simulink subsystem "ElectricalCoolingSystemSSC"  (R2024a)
settings: Solver=VariableStepAuto  StartTime=0.0  StopTime=10.0  RelTol=1e-3
undefined symbols (not defined in the file): BattTempInit, One, Pass, pipe, pump, radiator, T_env, tank, ThrmBatt1, ThrmBatt2, ThrmBatt3, ThrmBatt4, ThrmEM1, ThrmEM2, ThrmEM3, ThrmEM4, valve
libraries: fl_lib x109, SimscapeFluids_lib x7, nesl_utility_internal x6, autolibutils x2, nesl_utility x1, sdl_lib x1
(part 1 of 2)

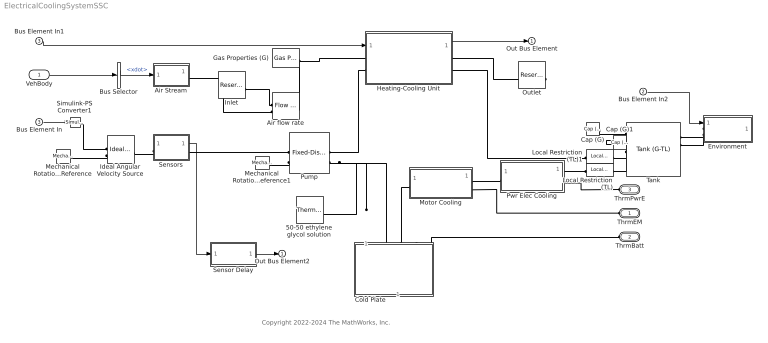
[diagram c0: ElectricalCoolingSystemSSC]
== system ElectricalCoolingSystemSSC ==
  note: Copyright 2022-2024 The MathWorks, Inc.
  VehBody : Inport
  Bus Element In2 : Inport  Port=2
  Bus Element In1 : Inport  Port=3
  Bus Element In : Inport  Port=3
  50-50 ethylene glycol solution : SimscapeFluids_lib/Thermal Liquid/Utilities/Thermal Liquid Properties (TL)  fluid_list=fluids.thermal_liquid.utilities.enum.thermal_liquid_fluid_list.ethylene_glycol  concentration_param_EG=fluids.thermal_liquid.utilities.enum.thermal_liquid_concentration.volume_fraction  concentration_param_PG=fluids.thermal_liquid.utilities.enum.thermal_liquid_concentration.volume_fraction  c_mass_SW=3.5e-3  c_mass_EG=0.1  c_mass_PG=0.1  c_mass_GL=0.1  c_vol_EG=0.5  c_vol_PG=0.1  beta_const_EG=2.1791 GPa  beta_const_PG=2.1791 GPa  beta_const_GL=2.1791 GPa  p_min_EG=0.01 MPa  p_min_PG=0.01 MPa  p_min_GL=0.01 MPa  p_max_EG=50 MPa  p_max_PG=50 MPa  p_max_GL=50 MPa  p_atm=0.101325 MPa  properties_range_check=simscape.enum.assert.action.error
  Air Stream : Subsystem
  Air flow rate : fl_lib/Gas/Sources/Flow Rate Source (G)  source_type=foundation.enum.constant_controlled.controlled  flow_type=foundation.enum.mass_volumetric_flow.mass  mass_flow=0 kg/s  volumetric_flow=0 m^3/s  volumetric_flow_conditions=foundation.enum.volumetric_flow_conditions.actual  p_std=0.101325 MPa  T_std=20 degC  power_spec=0  area_A=radiator.area_air m^2  area_B=radiator.area_air m^2
  Bus Selector : BusSelector  OutputSignals=BdyFrm.Cg.Vel.xdot
  Cap (G) : fl_lib/Gas/Elements/Cap (G)  p_specify=off  p_priority=None  p=0.101325 MPa  p_nominal_specify=off  p_nominal_value=1  p_nominal_unit=MPa  T_specify=off  T_priority=None  T=293.15 K  T_nominal_specify=off  T_nominal_value=1  T_nominal_unit=K
  Cap (G)1 : fl_lib/Gas/Elements/Cap (G)  p_specify=off  p_priority=None  p=0.101325 MPa  p_nominal_specify=off  p_nominal_value=1  p_nominal_unit=MPa  T_specify=off  T_priority=None  T=293.15 K  T_nominal_specify=off  T_nominal_value=1  T_nominal_unit=K
  Cold Plate : Subsystem  Variant=on  VariantControlMode=label  VariantControl=Choice  LabelModeActiveChoice=One-Pass
  Environment : Subsystem
  Gas Properties (G) : fl_lib/Gas/Utilities/Gas Properties (G)  gas_spec=1  R=0.287 kJ/kg/K  Z=1  T_ref=293.15 K  h_ref=420 kJ/kg  cp_ref=1 kJ/kg/K  mu_ref=18 s*uPa  k_ref=26 mW/m/K  T_TLU1=[150 : 10 : 200, 250 : 50 : 1000, 1500, 2000] K  h_TLU1=[275.264783730547; 285.377054177734; 295.474578903607; 305.560871069627; 315.638490783961; 325.709373787179; 376.008033649461; 426.297784741196; 476.678788323875; 527.253890684429; 578.12722735187; 629.395040865183; 681.137690131207; 733.415442873049; 786.267894376777; 839.715851152006; 893.764459999509; 948.406676876931; 1003.62653219711; 1059.40193232821; 1115.70691941005; 1172.51341226958; 1762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  cp_TLU1=[1.01211492398124; 1.01042105529234; 1.00914159006373; 1.00815898273273; 1.00739688341918; 1.00680484569075; 1.00554191216852; 1.00637389921747; 1.0092105862442; 1.01414404435034; 1.02111299587909; 1.02986878923959; 1.04003820504128; 1.05120320041448; 1.06296312852444; 1.07497111709439; 1.08694865668905; 1.0986858495625; 1.11003396604319; 1.12089493621399; 1.13121051694521; 1.14095251451866; 1.210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  mu_TLU1=[10.3766056544352; 10.9908682444892; 11.5932000841352; 12.1841060353213; 12.764067709023; 13.3335437107148; 16.038149065057; 18.5373404836509; 20.8671495114253; 23.0554226800681; 25.1239717991959; 27.0901379793485; 28.96790749834; 30.7687111230031; 32.5020036481173; 34.17569027566; 35.7964450415303; 37.3699520751368; 38.9010908824946; 40.3940804368247; 41.8525925389218; 43.279841956487; 56.3254722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  k_TLU1=[14.1517155766309; 15.0474512994325; 15.9300520513026; 16.7998749295306; 17.6573089963228; 18.5027588910197; 22.5644026699512; 26.384465676638; 30.0032801168886; 33.4532006033488; 36.7600619429332; 39.9446251241844; 43.0237448740114; 46.0112537033799; 48.9186234516389; 51.7554617696538; 54.5298878921773; 57.2488200454925; 59.9181976996146; 62.5431553064749; 65.128159527924; 67.6771186900213; 91.78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  T_TLU2=[150 : 10 : 200, 250 : 50 : 1000, 1500, 2000] K  p_TLU2=[0.001, 0.005, 0.01 : 0.01 : 0.1, 0.12, 0.15, 0.2, 0.5, 1, 2, 5, 10] MPa  rho_TLU2=[.0232262435294122, .116159536418799, .232389928446798, .465063671432694, .698022015548056, .931265751213184, 1.16479567270147, 1.39861257816015, 1.6327172696322, 1.86711055307826, 2.10179323839862, 2.33676613945539, 2.80758586416975, 3.5160126461103, 4.70263894299404, 11.983516436453, 24.7878864888476, 53.4753944012435, 188.202476404452, 488.088746553617; .0217743613495483, .108893511712, .217841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  s_TLU2=[4.51795188269071, 4.05581817155212, 3.85666832168988, 3.65733557342939, 3.54058125651975, 3.45763599951791, 3.39321600973057, 3.34051347760226, 3.2958969095816, 3.25719862711102, 3.22302043260479, 3.19240764614444, 3.13933271586112, 3.07416650003008, 2.98972303348322, 2.71525667312277, 2.4961408855038, 2.25200576011077, 1.78471429674036, 1.29090458888978; 4.58264139768585, 4.12053027678858, 3.921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  h_TLU2=[276.08088424589, 276.048494255671, 276.007989595737, 275.926922934925, 275.845779642901, 275.764559507019, 275.68326231383, 275.601887849085, 275.520435897725, 275.438906243879, 275.357298670861, 275.275612961165, 275.112006257597, 274.86600469197, 274.45440990197, 271.941510053176, 267.573991878308, 258.028969756929, 218.234362269026, 158.930370089034; 286.104280121225, 286.075386875978, 286.039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  cp_TLU2=[1.00234082589656, 1.00272486727657, 1.00320557010184, 1.0041691525775, 1.00513564892549, 1.00610507294701, 1.00707743852905, 1.00805275964505, 1.00903105035552, 1.01001232480866, 1.01099659724104, 1.01198388197822, 1.01396754611819, 1.01696599794404, 1.02202562270308, 1.05412155485561, 1.1152747482059, 1.27776397304517, 2.72714600163742, 2.84169679152775; 1.00233987250094, 1.0026582461868, 1.0030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  mu_TLU2=[10.3589401268092, 10.3596215490306, 10.3604759816291, 10.3621937105615, 10.3639232830336, 10.3656647294411, 10.367418080323, 10.3691833663632, 10.3709606183908, 10.3727498673813, 10.3745511444581, 10.3763644808926, 10.3800274576703, 10.3856131584654, 10.3951680979376, 10.4591651061333, 10.5933716881858, 10.987254253246, 14.2772531553238, 32.0640438449792; 10.9730737505367, 10.9737639649823, 10.97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  k_TLU2=[14.0836394676256, 14.0862942007498, 14.0896194596466, 14.0962928994967, 14.102997040872, 14.1097320212018, 14.1164979631452, 14.1232949816993, 14.1301231872323, 14.1369826870758, 14.143873586467, 14.1507959891554, 14.1647357143434, 14.1858841226196, 14.2217750346856, 14.4546939871274, 14.9161812046845, 16.179147415959, 25.804405174674, 52.7180018225101; 14.9842167167395, 14.9866891286677, 14.9897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  beta_TLU2=[.000999939063271047, .00499847620325299, .00999390291790365, .019975596477506, .0299450577879351, .0399022638252297, .0498471914323395, .0597798173190184, .0697001180617656, .0796080701037593, .0895036497547952, .0993868331912267, .119115915458133, .148615963978671, .197531539031374, .484259268054388, .934728751330763, 1.71724988255064, 2.82175958388315, 17.9919018393343; .000999950175637603, .00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  alpha_TLU2=[.00666792026017809, .00667293852525301, .00667922012518017, .00669181264110188, .00670444439920956, .0067171155853866, .00672982638662978, .00674257699105705, .00675536758791526, .00676819836758812, .00678106952160409, .00679398124264439, .00681992716233515, .00685915517876874, .00692537286982025, .00734607851757868, .00815022150220267, .0102947700145685, .0286130234990625, .0187953609548895; .00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  T_min_perfect=1 K  T_max_perfect=inf K  p_min_perfect=1e-6 MPa  p_max_perfect=inf MPa  T_range_flag=1  T_min_semiperfect=150 K  T_max_semiperfect=2000 K  p_min_semiperfect=1e-6 MPa  p_max_semiperfect=inf MPa  pT_region_flag=1  pT_validity_TLU2=ones(24, 20)  T_min_real=150 K  T_max_real=2000 K  p_min_real=0.001 MPa  p_max_real=10 MPa  p_atm=0.101325 MPa  properties_range_check=simscape.enum.assert.action.error  Mach_rev=0.001
  Heating-Cooling Unit : Subsystem
  Ideal Angular Velocity Source : fl_lib/Mechanical/Mechanical Sources/Ideal Angular Velocity Source
  Inlet : fl_lib/Gas/Elements/Reservoir (G)  pressure_spec=1  reservoir_pressure=0.101325 MPa  reservoir_temperature=EnvAirTempC degC  area_A=radiator.area_air m^2
  Local Restriction (TL) : fl_lib/Thermal Liquid/Elements/Local Restriction (TL)  restriction_type=foundation.enum.restriction_type.fixed  restriction_area=pipe.area/1.1 cm^2  min_area=1e-10 m^2  max_area=0.005 m^2  area=pipe.area cm^2  Cd=0.7  Re_c=12  pressure_recovery=simscape.enum.onoff.on
  Local Restriction (TL)1 : fl_lib/Thermal Liquid/Elements/Local Restriction (TL)  restriction_type=foundation.enum.restriction_type.fixed  restriction_area=pipe.area/1.1 cm^2  min_area=1e-10 m^2  max_area=0.005 m^2  area=pipe.area cm^2  Cd=0.7  Re_c=12  pressure_recovery=simscape.enum.onoff.on
  Mechanical Rotational Reference : fl_lib/Mechanical/Rotational Elements/Mechanical Rotational Reference
  Mechanical Rotational Reference1 : fl_lib/Mechanical/Rotational Elements/Mechanical Rotational Reference
  Motor Cooling : Subsystem  Tag=PublishSubsystem
  Outlet : fl_lib/Gas/Elements/Reservoir (G)  pressure_spec=1  reservoir_pressure=0.101325 MPa  reservoir_temperature=EnvAirTempC K  area_A=radiator.area_air m^2
  Pump : SimscapeFluids_lib/Thermal Liquid/Pumps & Motors/Fixed-Displacement Pump (TL)  loss_spec=1  displacement=pump.displacement cm^3/rev  omega_nominal=pump.omega rpm  p_nominal=1 MPa  mu_nominal=0.9 cP  vol_eff_nominal=0.92  mech_eff_nominal=1/(1 + (0.6)/(pump.displacement)*6.283185307179584 + (0.05)/(pump.displacement)/(1)*6.283185307179584)  no_load_torque=0.05 N*m  p_diff_eff_TLU=[.1, 1, 2] MPa  omega_eff_TLU=[25, 50, 100, 200, 300, 400] rad/s  vol_eff_TLU=[.816, .908, .954, .977, .981, .984; .325, .663, .831, .916, .925, .946; .137, .568, .78, .892, .893, .91]  mech_eff_TLU=[.996, .996, .996, .996, .996, .996; .988, .989, .989, .989, .989, .99; .981, .981, .982, .982, .983, .984]  p_diff_loss_TLU=[.1, 1, 2] MPa  omega_loss_TLU=[25, 50, 100, 200, 300, 400] rad/s  vol_loss_TLU=[.023, .023, .023, .023, .0285, .032; .0844, .0842, .0845, .084, .1125, .108; .1079, .108, .11, .108, .1605, .18] * 1e-3 m^3/s  mech_loss_TLU=[.002, .002, .002, .002, .002, .002; .0607, .0556, .0556, .0556, .0556, .0505; .1937, .1937, .1833, .1833, .1729, .1626] N*m  vol_eff_min=1e-3  vol_eff_max=1  mech_eff_min=1e-3  mech_eff_max=1  pressure_threshold=1e-3 MPa  omega_threshold=10 rad/s  area=pipe.area cm^2  supplied_range_check=0  pump_mode_check=simscape.enum.assert.action.none
  Pwr Elec Cooling : Subsystem
  Sensor Delay : Subsystem  mask{wc=10, InitCond=0, dataType=off}
      mask prompts: wc "Cutoff frequency, wc [rad/s]"; InitCond "Initial condition, InitCond [same as u]"; dataType "Enforce same input data type"
  Sensors : Subsystem
  Simulink-PS Converter1 : nesl_utility_internal/Simulink-PS Converter  PhysicalDomain=network_engine_domain  SubClassName=ps_input  LeftPortType=input  RightPortType=output  PseudoPeriodic=off  Frequencies=[]  NoiseDistribution=none  NoiseParameters=[]  Unit=rpm  AffineConversion=off  FilteringAndDerivatives=provide  SimscapeFilterOrder=1  InputFilterTimeConstant=0.001  UdotUserProvided=0
  Tank : SimscapeFluids_lib/Thermal Liquid/Tanks & Accumulators/Tank (G-TL)  num_inlet=6  volume_total=tank.volume l  volume_spec=1  tank_area=tank.area m^2  level_TLU=[0, 3, 5] m  volume_TLU=[0, 4, 6] m^3  inlet_areas_A1B1=[.01, .01] m^2  inlet_height_A2=0.1 m  inlet_area_A2=0.01 m^2  inlet_heights_A2B2=[0.0, 0.0] m  inlet_areas_A2B2=pipe.area*[1.0, 1.0] cm^2  inlet_heights_A2B2C2=[.1, .05, 0] m  inlet_areas_A2B2C2=[.01, .01, .01] m^2  inlet_heights_A2B2C2D2=0.1 * ones(1, 4) m  inlet_areas_A2B2C2D2=0.01 * ones(1, 4) m^2  inlet_heights_A2B2C2D2E2=0.1 * ones(1, 5) m  inlet_areas_A2B2C2D2E2=0.01 * ones(1, 5) m^2  inlet_heights_A2B2C2D2E2F2=0.07 * ones(1, 6) m  inlet_areas_A2B2C2D2E2F2=0.01 * ones(1, 6) m^2  capacity_check=1  max_liquid_capacity=tank.volume l  g=0 m/s^2  level_specify=on  level_priority=None  level=0.2 m  level_nominal_specify=off  level_nominal_value=1  level_nominal_unit=m  volume_liquid_specify=on  volume_liquid_priority=High  volume_liquid=5 l  volume_liquid_nominal_specify=off  volume_liquid_nominal_value=1  volume_liquid_nominal_unit=m^3  mass_liquid_specify=off  mass_liquid_priority=None  mass_liquid=5e+3 kg  mass_liquid_nominal_specify=off  mass_liquid_nominal_value=1  mass_liquid_nominal_unit=kg  T_liquid_specify=off  T_liquid_priority=High  T_liquid=293.15 K  T_liquid_nominal_specify=off  T_liquid_nominal_value=1  T_liquid_nominal_unit=K  p_gas_specify=off  p_gas_priority=High  p_gas=0.101325 MPa  p_gas_nominal_specify=off  p_gas_nominal_value=1  p_gas_nominal_unit=MPa  T_gas_specify=off  T_gas_priority=High  T_gas=293.15 K  T_gas_nominal_specify=off  T_gas_nominal_value=1  T_gas_nominal_unit=K  rho_gas_specify=off  rho_gas_priority=None  rho_gas=1.2 kg/m^3  rho_gas_nominal_specify=off  rho_gas_nominal_value=1  rho_gas_nominal_unit=kg/m^3
  ThrmEM : PMIOPort  Side=Left
  ThrmBatt : PMIOPort  Port=2  Side=Left
  ThrmPwrE : PMIOPort  Port=3  Side=Left
  Out Bus Element2 : Outport
  Out Bus Element : Outport
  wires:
  VehBody/1 -> Bus Selector/1
  Sensor Delay/1(y) -> Out Bus Element2/1
  Bus Element In/1 -> Simulink-PS Converter1/1
  Sensors/1(CoolPwr) -> Sensor Delay/1(u)
  Bus Element In1/1 -> Heating-Cooling Unit/1(ValveCmd)
  Bus Selector/1 -> Air Stream/1(V)  "<xdot>"
  Heating-Cooling Unit/1(CoolTemp) -> Out Bus Element/1
  Bus Element In2/1 -> Environment/1(AmbTmp)
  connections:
  Gas Properties (G)/RConn1 -- Heating-Cooling Unit/LConn1 -- Air flow rate/RConn1
  Pump/LConn2 -- 50-50 ethylene glycol solution/RConn1 -- Cold Plate/LConn1
  Cap (G)1/LConn1 -- Tank/LConn2
  Cap (G)/LConn1 -- Tank/LConn1
  Sensors/RConn1 -- Pump/RConn1
  Air flow rate/LConn1 -- Inlet/LConn1
  Pump/RConn2 -- Mechanical Rotational Reference1/LConn1
  Heating-Cooling Unit/RConn1 -- Outlet/LConn1
  Air flow rate/LConn2 -- Air Stream/RConn1
  Tank/LConn3 -- Local Restriction (TL)1/RConn1
  Environment/LConn1 -- Tank/RConn1
  Environment/LConn2 -- Tank/RConn2
  Local Restriction (TL)1/LConn1 -- Heating-Cooling Unit/RConn2
  Heating-Cooling Unit/LConn2 -- Pump/LConn1
  ThrmBatt/RConn1 -- Cold Plate/LConn3
  Sensors/LConn1 -- Ideal Angular Velocity Source/LConn1
  Simulink-PS Converter1/RConn1 -- Ideal Angular Velocity Source/RConn1
  Ideal Angular Velocity Source/RConn2 -- Mechanical Rotational Reference/LConn1
  Tank/LConn4 -- Local Restriction (TL)/RConn1
  Pwr Elec Cooling/RConn1 -- Local Restriction (TL)/LConn1
  Pwr Elec Cooling/RConn2 -- ThrmPwrE/RConn1
  Motor Cooling/RConn1 -- Pwr Elec Cooling/LConn1
  Cold Plate/LConn2 -- Motor Cooling/LConn1
  ThrmEM/RConn1 -- Motor Cooling/RConn2

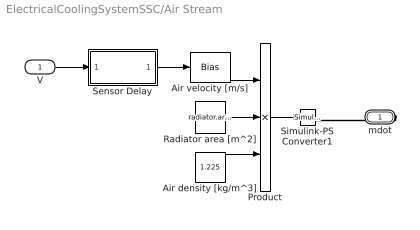
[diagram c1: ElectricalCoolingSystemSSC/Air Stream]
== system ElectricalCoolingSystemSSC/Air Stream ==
  V : Inport
  Air density [kg/m^3] : Constant  Value=1.225
  Air velocity [m/s] : Bias  Bias=5
  Product : Product  Inputs=3
  Radiator area [m^2] : Constant  Value=radiator.area_air
  Sensor Delay : Subsystem  mask{wc=100, InitCond=0, dataType=off}
      mask prompts: wc "Cutoff frequency, wc [rad/s]"; InitCond "Initial condition, InitCond [same as u]"; dataType "Enforce same input data type"
  Simulink-PS Converter1 : nesl_utility_internal/Simulink-PS Converter  PhysicalDomain=network_engine_domain  SubClassName=ps_input  LeftPortType=input  RightPortType=output  PseudoPeriodic=off  Frequencies=[]  NoiseDistribution=none  NoiseParameters=[]  Unit=kg/s  AffineConversion=off  FilteringAndDerivatives=provide  SimscapeFilterOrder=1  InputFilterTimeConstant=0.01  UdotUserProvided=0
  mdot : PMIOPort  Side=Right
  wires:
  V/1 -> Sensor Delay/1(u)
  Product/1 -> Simulink-PS Converter1/1
  Radiator area [m^2]/1 -> Product/2
  Air density [kg/m^3]/1 -> Product/3
  Air velocity [m/s]/1 -> Product/1
  Sensor Delay/1(y) -> Air velocity [m/s]/1
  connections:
  mdot/RConn1 -- Simulink-PS Converter1/RConn1

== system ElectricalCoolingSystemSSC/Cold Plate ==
  One-Pass : Subsystem  VariantControl=One-Pass
  Inlet : PMIOPort  Side=Left
  Outlet : PMIOPort  Port=2  Side=Left
  ThrmBatt : PMIOPort  Port=3  Side=Left

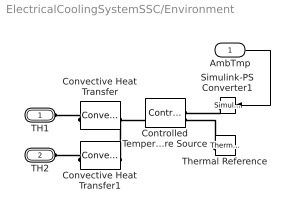
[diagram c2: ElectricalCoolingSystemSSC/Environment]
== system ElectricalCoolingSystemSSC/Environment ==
  AmbTmp : Inport
  Controlled Temperature Source : fl_lib/Thermal/Thermal Sources/Controlled Temperature Source
  Convective Heat Transfer : fl_lib/Thermal/Thermal Elements/Convective Heat Transfer  thermal_type=foundation.enum.constant_variable.constant  area=tank.area_wall/2 m^2  heat_tr_coeff=20 W/(m^2 * K)  min_heat_tr_coeff=1e-3 W/(K*m^2)  T_specify=off  T_priority=None  T=0 K  T_nominal_specify=off  T_nominal_value=1  T_nominal_unit=K  Q_specify=off  Q_priority=None  Q=0 W  Q_nominal_specify=off  Q_nominal_value=1  Q_nominal_unit=W
  Convective Heat Transfer1 : fl_lib/Thermal/Thermal Elements/Convective Heat Transfer  thermal_type=foundation.enum.constant_variable.constant  area=tank.area_wall/2 m^2  heat_tr_coeff=20 W/(m^2 * K)  min_heat_tr_coeff=1e-3 W/(K*m^2)  T_specify=off  T_priority=None  T=0 K  T_nominal_specify=off  T_nominal_value=1  T_nominal_unit=K  Q_specify=off  Q_priority=None  Q=0 W  Q_nominal_specify=off  Q_nominal_value=1  Q_nominal_unit=W
  Simulink-PS Converter1 : nesl_utility_internal/Simulink-PS Converter  PhysicalDomain=network_engine_domain  SubClassName=ps_input  LeftPortType=input  RightPortType=output  PseudoPeriodic=off  Frequencies=[]  NoiseDistribution=none  NoiseParameters=[]  Unit=K  AffineConversion=on  FilteringAndDerivatives=provide  SimscapeFilterOrder=1  InputFilterTimeConstant=0.001  UdotUserProvided=0
  Thermal Reference : fl_lib/Thermal/Thermal Elements/Thermal Reference
  TH1 : PMIOPort  Side=Left
  TH2 : PMIOPort  Port=2  Side=Left
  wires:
  AmbTmp/1 -> Simulink-PS Converter1/1
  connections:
  Thermal Reference/LConn1 -- Controlled Temperature Source/RConn2
  Simulink-PS Converter1/RConn1 -- Controlled Temperature Source/RConn1
  Convective Heat Transfer1/RConn1 -- Controlled Temperature Source/LConn1 -- Convective Heat Transfer/RConn1
  Convective Heat Transfer1/LConn1 -- TH2/RConn1
  Convective Heat Transfer/LConn1 -- TH1/RConn1

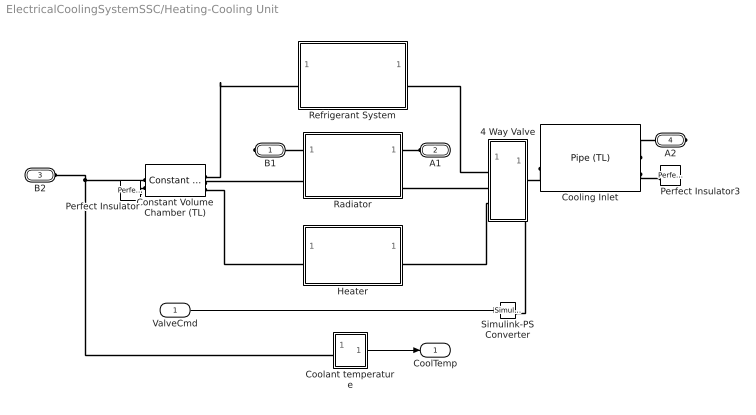
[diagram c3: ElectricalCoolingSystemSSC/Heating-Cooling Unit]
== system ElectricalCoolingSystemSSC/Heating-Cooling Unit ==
  ValveCmd : Inport
  4 Way Valve : Subsystem
  Constant Volume Chamber (TL) : fl_lib/Thermal Liquid/Elements/Constant Volume Chamber (TL)  volume=5 cm^3  num_ports=foundation.enum.num_ports.four  area_A=pipe.area m^2  area_B=pipe.area*10 m^2  area_C=pipe.area m^2  area_D=pipe.area m^2  p_I_specify=off  p_I_priority=High  p_I=0.101325 MPa  p_I_nominal_specify=off  p_I_nominal_value=1  p_I_nominal_unit=MPa  T_I_specify=on  T_I_priority=High  T_I=BattTempInit degC  T_I_nominal_specify=off  T_I_nominal_value=1  T_I_nominal_unit=K  u_I_specify=off  u_I_priority=None  u_I=83.90600000000001 kJ/kg  u_I_nominal_specify=off  u_I_nominal_value=1  u_I_nominal_unit=kJ/kg  rho_I_specify=off  rho_I_priority=None  rho_I=998.21 kg/m^3  rho_I_nominal_specify=off  rho_I_nominal_value=1  rho_I_nominal_unit=kg/m^3
  Coolant temperature : Subsystem
  Cooling Inlet : fl_lib/Thermal Liquid/Elements/Pipe (TL)  length=0.75 m  area=pipe.area cm^2  Dh=pipe.Dh cm  length_add=0 m  roughness=15e-6 m  Re_lam=2000  Re_tur=4000  shape_factor=64  Nu_lam=3.66  dynamic_compressibility=simscape.enum.onoff.off  inertia=simscape.enum.onoff.off  p0=0.101325 MPa  T0=BattTempInit degC  mdot0=0 kg/s
  Heater : Subsystem
  Perfect Insulator : fl_lib/Thermal/Thermal Elements/Perfect Insulator  T_specify=off  T_priority=None  T=0 K  T_nominal_specify=off  T_nominal_value=1  T_nominal_unit=K
  Perfect Insulator3 : fl_lib/Thermal/Thermal Elements/Perfect Insulator  T_specify=off  T_priority=None  T=0 K  T_nominal_specify=off  T_nominal_value=1  T_nominal_unit=K
  Radiator : Subsystem
  Refrigerant System : Subsystem
  Simulink-PS Converter : nesl_utility_internal/Simulink-PS Converter  PhysicalDomain=network_engine_domain  SubClassName=ps_input  LeftPortType=input  RightPortType=output  PseudoPeriodic=off  Frequencies=[]  NoiseDistribution=none  NoiseParameters=[]  Unit=mm  AffineConversion=off  FilteringAndDerivatives=provide  SimscapeFilterOrder=1  InputFilterTimeConstant=0.001  UdotUserProvided=0
  B1 : PMIOPort  Side=Right
  A1 : PMIOPort  Port=2  Side=Left
  B2 : PMIOPort  Port=3  Side=Left
  A2 : PMIOPort  Port=4  Side=Right
  CoolTemp : Outport
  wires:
  ValveCmd/1 -> Simulink-PS Converter/1
  Coolant temperature/1(T) -> CoolTemp/1
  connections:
  Simulink-PS Converter/RConn1 -- 4 Way Valve/RConn2
  Perfect Insulator/LConn1 -- Constant Volume Chamber (TL)/LConn2
  Cooling Inlet/LConn2 -- Perfect Insulator3/LConn1
  Constant Volume Chamber (TL)/RConn1 -- Refrigerant System/LConn1
  Radiator/RConn2 -- 4 Way Valve/LConn2
  Cooling Inlet/RConn1 -- 4 Way Valve/RConn1
  Cooling Inlet/LConn1 -- A2/RConn1
  Radiator/RConn1 -- A1/RConn1
  Refrigerant System/RConn1 -- 4 Way Valve/LConn1
  Radiator/LConn1 -- B1/RConn1
  Constant Volume Chamber (TL)/RConn3 -- Heater/LConn1
  Constant Volume Chamber (TL)/LConn1 -- Coolant temperature/LConn1 -- B2/RConn1
  4 Way Valve/LConn3 -- Heater/RConn1
  Constant Volume Chamber (TL)/RConn2 -- Radiator/LConn2

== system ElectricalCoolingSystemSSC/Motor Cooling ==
  Cooling Assembly : Subsystem  Variant=on  VariantControl=Cooling Assembly
  Simscape Bus1 : SimscapeBus  HierarchyStrings=ThrmEM4;ThrmEM3;ThrmEM2;ThrmEM1
  A : PMIOPort  Side=Left
  B : PMIOPort  Port=2  Side=Right
  ThrmEM : PMIOPort  Port=3  Side=Right
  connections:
  Simscape Bus1/LConn1 -- Cooling Assembly/RConn2
  Simscape Bus1/LConn2 -- Cooling Assembly/RConn3
  Simscape Bus1/LConn3 -- Cooling Assembly/RConn4
  Simscape Bus1/LConn4 -- Cooling Assembly/RConn5
  B/RConn1 -- Cooling Assembly/RConn1
  A/RConn1 -- Cooling Assembly/LConn1
  ThrmEM/RConn1 -- Simscape Bus1/RConn1

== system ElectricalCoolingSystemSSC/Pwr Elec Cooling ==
  Cooling Jacket1 : Subsystem
  Pipe (TL) : fl_lib/Thermal Liquid/Elements/Pipe (TL)  length=pipe.length cm  area=pipe.area cm^2  Dh=pipe.Dh cm  length_add=0 m  roughness=15e-6 m  Re_lam=2000  Re_tur=4000  shape_factor=64  Nu_lam=3.66  dynamic_compressibility=simscape.enum.onoff.off  inertia=simscape.enum.onoff.off  p0=0.101325 MPa  T0=BattTempInit degC  mdot0=0 kg/s
  Simscape Bus3 : SimscapeBus  HierarchyStrings=ThrmPwrE1
  A : PMIOPort  Side=Left
  B : PMIOPort  Port=2  Side=Right
  ThrmPwrE : PMIOPort  Port=3  Side=Right
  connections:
  Pipe (TL)/RConn1 -- B/RConn1
  Pipe (TL)/LConn1 -- A/RConn1
  Pipe (TL)/LConn2 -- Cooling Jacket1/LConn1
  Simscape Bus3/RConn1 -- ThrmPwrE/RConn1
  Simscape Bus3/LConn1 -- Cooling Jacket1/RConn1

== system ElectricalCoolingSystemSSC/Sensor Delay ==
  u : Inport
  Cont LPF IC : autolibutils/Cont LPF IC  wc=wc  aMode=1  dataType=off
  Initial Condition : Constant  Value=InitCond  SampleTime=-1
  y : Outport
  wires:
  Initial Condition/1 -> Cont LPF IC/2
  u/1 -> Cont LPF IC/1
  Cont LPF IC/1 -> y/1

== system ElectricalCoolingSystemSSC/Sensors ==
  Add : Sum
  Mechanical Rotational Reference : fl_lib/Mechanical/Rotational Elements/Mechanical Rotational Reference
  PS-Simulink Converter : nesl_utility/PS-Simulink Converter  PhysicalDomain=network_engine_domain  SubClassName=ps_output  LeftPortType=input  RightPortType=output  PseudoPeriodic=off  Frequencies=[]  VectorFormat=inherit  Unit=inherit  AffineConversion=off
  Rotational Power Sensor : sdl_lib/Sensors/Rotational Power Sensor  measurement_type=sdl.enum.rotationalPowerSensorType.instantaneous  averaging_period=1 s  max_frequency=1000 Hz  max_speed=1000 rpm
  R : PMIOPort  Side=Left
  pump : PMIOPort  Port=2  Side=Right
  CoolPwr : Outport
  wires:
  Add/1 -> CoolPwr/1
  PS-Simulink Converter/1 -> Add/2  "PumpPwr"
  [CmpPwr] -> Add/1
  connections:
  Rotational Power Sensor/LConn3 -- Mechanical Rotational Reference/LConn1
  pump/RConn1 -- Rotational Power Sensor/LConn2
  Rotational Power Sensor/RConn1 -- PS-Simulink Converter/LConn1
  Rotational Power Sensor/LConn1 -- R/RConn1

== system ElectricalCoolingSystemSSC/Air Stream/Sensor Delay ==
  u : Inport
  Cont LPF IC : autolibutils/Cont LPF IC  wc=wc  aMode=1  dataType=off
  Initial Condition : Constant  Value=InitCond  SampleTime=-1
  y : Outport
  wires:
  Initial Condition/1 -> Cont LPF IC/2
  u/1 -> Cont LPF IC/1
  Cont LPF IC/1 -> y/1

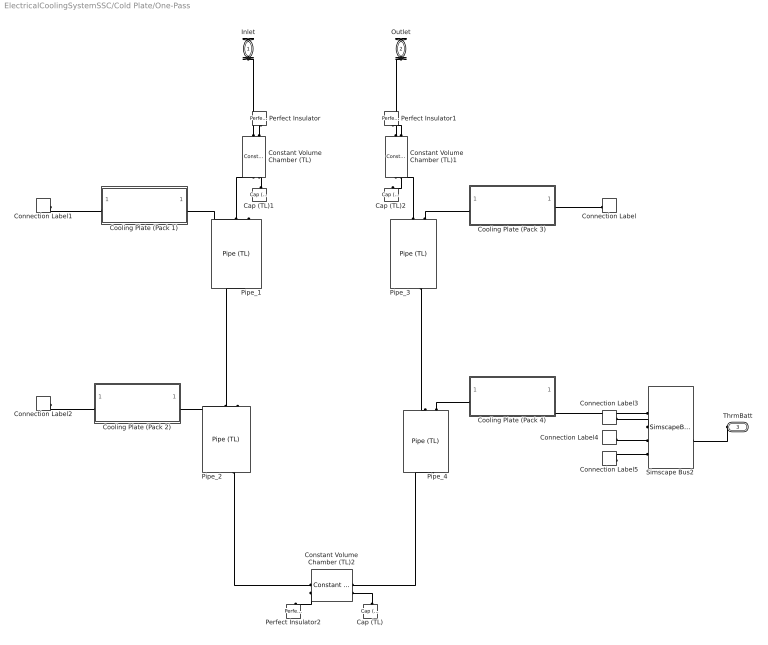
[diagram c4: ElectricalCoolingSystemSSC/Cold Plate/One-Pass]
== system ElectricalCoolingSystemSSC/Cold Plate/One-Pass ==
  Cap (TL) : fl_lib/Thermal Liquid/Elements/Cap (TL)  p_specify=off  p_priority=None  p=0.101325 MPa  p_nominal_specify=off  p_nominal_value=1  p_nominal_unit=MPa  T_specify=off  T_priority=None  T=293.15 K  T_nominal_specify=off  T_nominal_value=1  T_nominal_unit=K
  Cap (TL)1 : fl_lib/Thermal Liquid/Elements/Cap (TL)  p_specify=off  p_priority=None  p=0.101325 MPa  p_nominal_specify=off  p_nominal_value=1  p_nominal_unit=MPa  T_specify=off  T_priority=None  T=293.15 K  T_nominal_specify=off  T_nominal_value=1  T_nominal_unit=K
  Cap (TL)2 : fl_lib/Thermal Liquid/Elements/Cap (TL)  p_specify=off  p_priority=None  p=0.101325 MPa  p_nominal_specify=off  p_nominal_value=1  p_nominal_unit=MPa  T_specify=off  T_priority=None  T=293.15 K  T_nominal_specify=off  T_nominal_value=1  T_nominal_unit=K
  Connection Label : ConnectionLabel  Label=Pack3
  Connection Label1 : ConnectionLabel  Label=Pack1
  Connection Label2 : ConnectionLabel  Label=Pack2
  Connection Label3 : ConnectionLabel  Label=Pack3
  Connection Label4 : ConnectionLabel  Label=Pack2
  Connection Label5 : ConnectionLabel  Label=Pack1
  Constant Volume Chamber (TL) : fl_lib/Thermal Liquid/Elements/Constant Volume Chamber (TL)  volume=0.001 m^3  num_ports=foundation.enum.num_ports.three  area_A=3 cm^2  area_B=3 cm^2  area_C=3 cm^2  area_D=0.01 m^2  p_I_specify=off  p_I_priority=High  p_I=0.101325 MPa  p_I_nominal_specify=off  p_I_nominal_value=1  p_I_nominal_unit=MPa  T_I_specify=on  T_I_priority=High  T_I=BattTempInit degC  T_I_nominal_specify=off  T_I_nominal_value=1  T_I_nominal_unit=K  u_I_specify=off  u_I_priority=None  u_I=83.90600000000001 kJ/kg  u_I_nominal_specify=off  u_I_nominal_value=1  u_I_nominal_unit=kJ/kg  rho_I_specify=off  rho_I_priority=None  rho_I=998.21 kg/m^3  rho_I_nominal_specify=off  rho_I_nominal_value=1  rho_I_nominal_unit=kg/m^3
  Constant Volume Chamber (TL)1 : fl_lib/Thermal Liquid/Elements/Constant Volume Chamber (TL)  volume=0.001 m^3  num_ports=foundation.enum.num_ports.three  area_A=3 cm^2  area_B=3 cm^2  area_C=3 cm^2  area_D=0.01 m^2  p_I_specify=off  p_I_priority=High  p_I=0.101325 MPa  p_I_nominal_specify=off  p_I_nominal_value=1  p_I_nominal_unit=MPa  T_I_specify=on  T_I_priority=High  T_I=BattTempInit degC  T_I_nominal_specify=off  T_I_nominal_value=1  T_I_nominal_unit=K  u_I_specify=off  u_I_priority=None  u_I=83.90600000000001 kJ/kg  u_I_nominal_specify=off  u_I_nominal_value=1  u_I_nominal_unit=kJ/kg  rho_I_specify=off  rho_I_priority=None  rho_I=998.21 kg/m^3  rho_I_nominal_specify=off  rho_I_nominal_value=1  rho_I_nominal_unit=kg/m^3
  Constant Volume Chamber (TL)2 : fl_lib/Thermal Liquid/Elements/Constant Volume Chamber (TL)  volume=0.001 m^3  num_ports=foundation.enum.num_ports.three  area_A=3 cm^2  area_B=3 cm^2  area_C=3 cm^2  area_D=0.01 m^2  p_I_specify=off  p_I_priority=High  p_I=0.101325 MPa  p_I_nominal_specify=off  p_I_nominal_value=1  p_I_nominal_unit=MPa  T_I_specify=on  T_I_priority=High  T_I=BattTempInit degC  T_I_nominal_specify=off  T_I_nominal_value=1  T_I_nominal_unit=K  u_I_specify=off  u_I_priority=None  u_I=83.90600000000001 kJ/kg  u_I_nominal_specify=off  u_I_nominal_value=1  u_I_nominal_unit=kJ/kg  rho_I_specify=off  rho_I_priority=None  rho_I=998.21 kg/m^3  rho_I_nominal_specify=off  rho_I_nominal_value=1  rho_I_nominal_unit=kg/m^3
  Cooling Plate (Pack 1) : Subsystem
  Cooling Plate (Pack 2) : Subsystem
  Cooling Plate (Pack 3) : Subsystem
  Cooling Plate (Pack 4) : Subsystem
  Perfect Insulator : fl_lib/Thermal/Thermal Elements/Perfect Insulator  T_specify=off  T_priority=None  T=0 K  T_nominal_specify=off  T_nominal_value=1  T_nominal_unit=K
  Perfect Insulator1 : fl_lib/Thermal/Thermal Elements/Perfect Insulator  T_specify=off  T_priority=None  T=0 K  T_nominal_specify=off  T_nominal_value=1  T_nominal_unit=K
  Perfect Insulator2 : fl_lib/Thermal/Thermal Elements/Perfect Insulator  T_specify=off  T_priority=None  T=0 K  T_nominal_specify=off  T_nominal_value=1  T_nominal_unit=K
  Pipe_{1..4} (4 alike) : fl_lib/Thermal Liquid/Elements/Pipe (TL)  length=1.5 m  area=3*2 cm^2  Dh=0.92*sqrt(2) cm  length_add=0 m  roughness=15e-6 m  Re_lam=2000  Re_tur=4000  shape_factor=64  Nu_lam=3.66  dynamic_compressibility=simscape.enum.onoff.off  inertia=simscape.enum.onoff.off  p0=0.101325 MPa  T0=BattTempInit degC  mdot0=0 kg/s
  Simscape Bus2 : SimscapeBus  HierarchyStrings=ThrmBatt4;ThrmBatt3;ThrmBatt2;ThrmBatt1
  Inlet : PMIOPort  Side=Left
  Outlet : PMIOPort  Port=2  Side=Left
  ThrmBatt : PMIOPort  Port=3  Side=Left
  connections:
  ThrmBatt/RConn1 -- Simscape Bus2/RConn1
  Simscape Bus2/LConn2 -- Connection Label3/LConn1
  Simscape Bus2/LConn3 -- Connection Label4/LConn1
  Connection Label5/LConn1 -- Simscape Bus2/LConn4
  Constant Volume Chamber (TL)/LConn2 -- Perfect Insulator/LConn1
  Pipe_1/LConn1 -- Constant Volume Chamber (TL)/RConn1
  Constant Volume Chamber (TL)2/LConn2 -- Perfect Insulator2/LConn1
  Constant Volume Chamber (TL)2/RConn1 -- Pipe_4/RConn1
  Pipe_3/RConn1 -- Pipe_4/LConn1
  Cooling Plate (Pack 4)/RConn1 -- Simscape Bus2/LConn1
  Cooling Plate (Pack 3)/RConn1 -- Connection Label/LConn1
  Cooling Plate (Pack 2)/LConn1 -- Pipe_2/LConn2
  Cooling Plate (Pack 1)/LConn1 -- Pipe_1/LConn2
  Pipe_4/LConn2 -- Cooling Plate (Pack 4)/LConn1
  Pipe_3/LConn2 -- Cooling Plate (Pack 3)/LConn1
  Pipe_3/LConn1 -- Constant Volume Chamber (TL)1/RConn1
  Pipe_2/LConn1 -- Pipe_1/RConn1
  Connection Label2/LConn1 -- Cooling Plate (Pack 2)/RConn1
  Connection Label1/LConn1 -- Cooling Plate (Pack 1)/RConn1
  Constant Volume Chamber (TL)1/LConn1 -- Outlet/RConn1
  Constant Volume Chamber (TL)1/LConn2 -- Perfect Insulator1/LConn1
  Constant Volume Chamber (TL)/LConn1 -- Inlet/RConn1
  Pipe_2/RConn1 -- Constant Volume Chamber (TL)2/LConn1
  Cap (TL)/LConn1 -- Constant Volume Chamber (TL)2/RConn2
  Cap (TL)1/LConn1 -- Constant Volume Chamber (TL)/RConn2
  Constant Volume Chamber (TL)1/RConn2 -- Cap (TL)2/LConn1

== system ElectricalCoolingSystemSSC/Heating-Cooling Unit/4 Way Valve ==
  Variable Area Orifice (TL) : SimscapeFluids_lib/Thermal Liquid/Valves & Orifices/Orifice (TL)  orifice_type=foundation.enum.constant_variable.variable  constant_orifice_spec=fluids.thermal_liquid.valves.enum.ConstantOrificeSpec.Area  variable_orifice_spec=2  orifice_area_constant=1e-3 m^2  p_diff_TLU_constant=[-4, -3, -2, -1, -.5, 0, .5, 1, 2, 3, 4] MPa  vol_flow_TLU_constant=[-2.44, -2.12, -1.68, -1.22, -.84, 0, .85, 1.21, 1.7, 2.09, 2.41] .* 1e-3 m^3/s  mdot_TLU_constant=[-2.44, -2.12, -1.68, -1.22, -.84, 0, .85, 1.21, 1.7, 2.09, 2.41] kg/s  S_min=5e-06 mm  del_S=0.004999995 m  open_orientation=1  area_max=1e-4 m^2  area_leak=1e-10 m^2  S_TLU=[2 3] mm  orifice_area_TLU=[valve.opening, valve.area_leak] cm^2  Cd=0.7  Re_c=12  smoothing_factor=0.01  pressure_recovery=1  S_flow_TLU=[-2 0 2 5 15] mm  p_diff_TLU=[-.1, .3, .5, .7] MPa  vol_flow_TLU=1e-3 * [1.7e-05, 2e-05, 2.6e-05; .0035, .0045, .0053; .7, .9, 1.06; 1.96, 2.5, 3; 6, 7.7, 9.13] m^3/s  mdot_TLU=[-1e-05, 1.7e-05, 2e-05, 2.6e-05; -.002, .0035, .0045, .0053; -.4, .7, .9, 1.06; -1.13, 1.96, 2.5, 3; -3.45, 6, 7.7, 9.13] kg/s  T_ref_in=293.15 K  p_ref_in=0.101325 MPa  area=valve.area cm^2
  Variable Area Orifice (TL)1 : SimscapeFluids_lib/Thermal Liquid/Valves & Orifices/Orifice (TL)  orifice_type=foundation.enum.constant_variable.variable  constant_orifice_spec=fluids.thermal_liquid.valves.enum.ConstantOrificeSpec.Area  variable_orifice_spec=fluids.thermal_liquid.valves.enum.orifice_spec.table1D_area_opening  orifice_area_constant=1e-3 m^2  p_diff_TLU_constant=[-4, -3, -2, -1, -.5, 0, .5, 1, 2, 3, 4] MPa  vol_flow_TLU_constant=[-2.44, -2.12, -1.68, -1.22, -.84, 0, .85, 1.21, 1.7, 2.09, 2.41] .* 1e-3 m^3/s  mdot_TLU_constant=[-2.44, -2.12, -1.68, -1.22, -.84, 0, .85, 1.21, 1.7, 2.09, 2.41] kg/s  S_min=5e-06 mm  del_S=0.004999995 m  open_orientation=simscape.enum.posneg.positive  area_max=1e-4 m^2  area_leak=1e-10 m^2  S_TLU=[2 3 6 7] mm  orifice_area_TLU=[valve.area_leak, valve.opening, valve.opening, valve.area_leak] cm^2  Cd=0.7  Re_c=12  smoothing_factor=0.01  pressure_recovery=simscape.enum.onoff.on  S_flow_TLU=[-2 0 2 5 15] mm  p_diff_TLU=[-.1, .3, .5, .7] MPa  vol_flow_TLU=1e-3 * [1.7e-05, 2e-05, 2.6e-05; .0035, .0045, .0053; .7, .9, 1.06; 1.96, 2.5, 3; 6, 7.7, 9.13] m^3/s  mdot_TLU=[-1e-05, 1.7e-05, 2e-05, 2.6e-05; -.002, .0035, .0045, .0053; -.4, .7, .9, 1.06; -1.13, 1.96, 2.5, 3; -3.45, 6, 7.7, 9.13] kg/s  T_ref_in=293.15 K  p_ref_in=0.101325 MPa  area=valve.area cm^2
  Variable Area Orifice (TL)2 : SimscapeFluids_lib/Thermal Liquid/Valves & Orifices/Orifice (TL)  orifice_type=foundation.enum.constant_variable.variable  constant_orifice_spec=fluids.thermal_liquid.valves.enum.ConstantOrificeSpec.Area  variable_orifice_spec=fluids.thermal_liquid.valves.enum.orifice_spec.table1D_area_opening  orifice_area_constant=1e-3 m^2  p_diff_TLU_constant=[-4, -3, -2, -1, -.5, 0, .5, 1, 2, 3, 4] MPa  vol_flow_TLU_constant=[-2.44, -2.12, -1.68, -1.22, -.84, 0, .85, 1.21, 1.7, 2.09, 2.41] .* 1e-3 m^3/s  mdot_TLU_constant=[-2.44, -2.12, -1.68, -1.22, -.84, 0, .85, 1.21, 1.7, 2.09, 2.41] kg/s  S_min=5e-06 mm  del_S=0.004999995 m  open_orientation=simscape.enum.posneg.positive  area_max=1e-4 m^2  area_leak=1e-10 m^2  S_TLU=[6 7] mm  orifice_area_TLU=[valve.area_leak, valve.opening] cm^2  Cd=0.7  Re_c=12  smoothing_factor=0.01  pressure_recovery=simscape.enum.onoff.on  S_flow_TLU=[-2 0 2 5 15] mm  p_diff_TLU=[-.1, .3, .5, .7] MPa  vol_flow_TLU=1e-3 * [1.7e-05, 2e-05, 2.6e-05; .0035, .0045, .0053; .7, .9, 1.06; 1.96, 2.5, 3; 6, 7.7, 9.13] m^3/s  mdot_TLU=[-1e-05, 1.7e-05, 2e-05, 2.6e-05; -.002, .0035, .0045, .0053; -.4, .7, .9, 1.06; -1.13, 1.96, 2.5, 3; -3.45, 6, 7.7, 9.13] kg/s  T_ref_in=293.15 K  p_ref_in=0.101325 MPa  area=valve.area cm^2
  T1 : PMIOPort  Side=Left
  A : PMIOPort  Port=2  Side=Right
  T2 : PMIOPort  Port=3  Side=Left
  T3 : PMIOPort  Port=4  Side=Left
  S : PMIOPort  Port=5  Side=Right
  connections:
  Variable Area Orifice (TL)1/RConn1 -- T2/RConn1
  Variable Area Orifice (TL)2/RConn1 -- T3/RConn1
  Variable Area Orifice (TL)/RConn1 -- T1/RConn1
  Variable Area Orifice (TL)/LConn1 -- Variable Area Orifice (TL)1/LConn1 -- A/RConn1 -- Variable Area Orifice (TL)2/LConn1
  Variable Area Orifice (TL)/LConn2 -- S/RConn1 -- Variable Area Orifice (TL)2/LConn2 -- Variable Area Orifice (TL)1/LConn2

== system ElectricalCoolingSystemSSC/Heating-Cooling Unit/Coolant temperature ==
  Absolute Reference (TL) : fl_lib/Thermal Liquid/Elements/Absolute Reference (TL)
  PS-Simulink Converter : nesl_utility_internal/PS-Simulink Converter  PhysicalDomain=network_engine_domain  SubClassName=ps_output  LeftPortType=input  RightPortType=output  PseudoPeriodic=off  Frequencies=[]  VectorFormat=1-D array  Unit=K  AffineConversion=on
  Pressure & Temperature Sensor (TL) : fl_lib/Thermal Liquid/Sensors/Pressure & Temperature Sensor (TL)  reference=foundation.enum.MeasurementReference.difference  pressure=false  pressure_spec=foundation.enum.PressureMeasementSpec.Absolute  temperature=true
  A : PMIOPort  Side=Left
  T : Outport  VectorParamsAs1DForOutWhenUnconnected=off
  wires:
  PS-Simulink Converter/1 -> T/1
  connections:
  PS-Simulink Converter/LConn1 -- Pressure & Temperature Sensor (TL)/RConn2
  Pressure & Temperature Sensor (TL)/RConn1 -- Absolute Reference (TL)/LConn1
  Pressure & Temperature Sensor (TL)/LConn1 -- A/RConn1

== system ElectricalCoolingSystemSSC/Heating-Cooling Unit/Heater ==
  Controlled Temperature Source1 : fl_lib/Thermal/Thermal Sources/Controlled Temperature Source
  Heater Temperature : Subsystem  mask{T_heat=303}
      mask prompts: T_heat "Heater nominal temperature (K)"
  Mass & Energy Flow Rate Sensor (TL) : fl_lib/Thermal Liquid/Sensors/Flow Rate Sensor (TL)  mass_flow_measure=true  volumetric_flow_measure=false  energy_flow_measure=true
  Pipe (TL) : fl_lib/Thermal Liquid/Elements/Pipe (TL)  length=pipe.length cm  area=pipe.area cm^2  Dh=pipe.Dh cm  length_add=0 m  roughness=15e-6 m  Re_lam=2000  Re_tur=4000  shape_factor=64  Nu_lam=3.66  dynamic_compressibility=simscape.enum.onoff.off  inertia=simscape.enum.onoff.off  p0=0.101325 MPa  T0=BattTempInit degC  mdot0=0 kg/s
  Thermal Reference1 : fl_lib/Thermal/Thermal Elements/Thermal Reference
  B : PMIOPort  Side=Left
  A : PMIOPort  Port=2  Side=Right
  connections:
  Controlled Temperature Source1/LConn1 -- Pipe (TL)/LConn2
  Pipe (TL)/LConn1 -- Mass & Energy Flow Rate Sensor (TL)/RConn1
  Pipe (TL)/RConn1 -- B/RConn1
  Thermal Reference1/LConn1 -- Controlled Temperature Source1/RConn2
  Mass & Energy Flow Rate Sensor (TL)/LConn1 -- A/RConn1
  Heater Temperature/LConn1 -- Mass & Energy Flow Rate Sensor (TL)/RConn2
  Controlled Temperature Source1/RConn1 -- Heater Temperature/RConn1

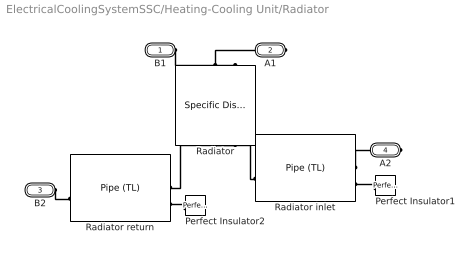
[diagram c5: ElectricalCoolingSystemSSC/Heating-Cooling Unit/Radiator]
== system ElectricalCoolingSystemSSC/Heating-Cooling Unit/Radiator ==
  Perfect Insulator1 : fl_lib/Thermal/Thermal Elements/Perfect Insulator  T_specify=off  T_priority=None  T=0 K  T_nominal_specify=off  T_nominal_value=1  T_nominal_unit=K
  Perfect Insulator2 : fl_lib/Thermal/Thermal Elements/Perfect Insulator  T_specify=off  T_priority=None  T=0 K  T_nominal_specify=off  T_nominal_value=1  T_nominal_unit=K
  Radiator : SimscapeFluids_lib/Heat Exchangers/Thermal Liquid - Gas/Specific Dissipation Heat Exchanger (G-TL)  mdot1_TLU=radiator.mdot_air kg/s  mdot2_TLU=radiator.mdot_liquid kg/s  SD_TLU=radiator.SD kW/K  Q_check=simscape.enum.assert.action.none  mdot_dp_TLU_1=radiator.mdot_air kg/s  p_diff_TLU_1=radiator.dp_air MPa  T_ref_in_1=293.15 K  p_ref_in_1=0.101325 MPa  mdot_threshold_1=1e-6 kg/s  gas_volume_1=radiator.volume_air m^3  area_1=radiator.area_air m^2  mdot_dp_TLU_2=radiator.mdot_liquid kg/s  p_diff_TLU_2=radiator.dp_liquid MPa  T_ref_in_2=293.15 K  p_ref_in_2=0.101325 MPa  mdot_threshold_2=1e-3 kg/s  liquid_volume_2=radiator.volume_liquid m^3  area_2=pipe.area cm^2  T0_1=BattTempInit degC  p0_1=0.105081 %0.101325 MPa  dynamic_compressibility_2=simscape.enum.onoff.on  T0_2=BattTempInit degC  p0_2=0.105081 %0.101325 MPa
  Radiator inlet : fl_lib/Thermal Liquid/Elements/Pipe (TL)  length=0.25 m  area=pipe.area cm^2  Dh=pipe.Dh cm  length_add=0 m  roughness=15e-6 m  Re_lam=2000  Re_tur=4000  shape_factor=64  Nu_lam=3.66  dynamic_compressibility=simscape.enum.onoff.off  inertia=simscape.enum.onoff.off  p0=0.101325 MPa  T0=BattTempInit degC  mdot0=0 kg/s
  Radiator return : fl_lib/Thermal Liquid/Elements/Pipe (TL)  length=0.25 m  area=pipe.area cm^2  Dh=pipe.Dh cm  length_add=0 m  roughness=15e-6 m  Re_lam=2000  Re_tur=4000  shape_factor=64  Nu_lam=3.66  dynamic_compressibility=simscape.enum.onoff.off  inertia=simscape.enum.onoff.off  p0=0.101325 MPa  T0=BattTempInit degC  mdot0=0 kg/s
  B1 : PMIOPort  Side=Left
  A1 : PMIOPort  Port=2  Side=Right
  B2 : PMIOPort  Port=3  Side=Left
  A2 : PMIOPort  Port=4  Side=Right
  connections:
  Perfect Insulator2/LConn1 -- Radiator return/LConn2
  Perfect Insulator1/LConn1 -- Radiator inlet/LConn2
  Radiator inlet/RConn1 -- Radiator/RConn1
  Radiator inlet/LConn1 -- A2/RConn1
  Radiator return/LConn1 -- Radiator/RConn2
  Radiator/LConn1 -- A1/RConn1
  B1/RConn1 -- Radiator/LConn2
  B2/RConn1 -- Radiator return/RConn1

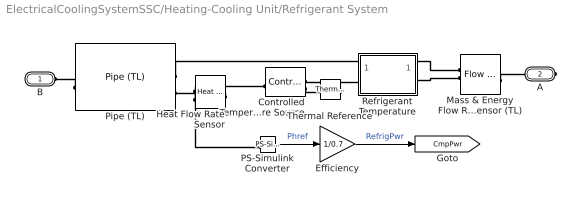
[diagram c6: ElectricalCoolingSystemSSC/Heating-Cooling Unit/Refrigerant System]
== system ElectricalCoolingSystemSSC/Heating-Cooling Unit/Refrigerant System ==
  Controlled Temperature Source : fl_lib/Thermal/Thermal Sources/Controlled Temperature Source
  Efficiency : Gain  Gain=1/0.7
  Heat Flow Rate Sensor : fl_lib/Thermal/Thermal Sensors/Heat Flow Rate Sensor
  Mass & Energy Flow Rate Sensor (TL) : fl_lib/Thermal Liquid/Sensors/Flow Rate Sensor (TL)  mass_flow_measure=true  volumetric_flow_measure=false  energy_flow_measure=true
  PS-Simulink Converter : nesl_utility_internal/PS-Simulink Converter  PhysicalDomain=network_engine_domain  SubClassName=ps_output  LeftPortType=input  RightPortType=output  PseudoPeriodic=off  Frequencies=[]  VectorFormat=1-D array  Unit=kW  AffineConversion=off
  Pipe (TL) : fl_lib/Thermal Liquid/Elements/Pipe (TL)  length=pipe.length cm  area=pipe.area*10 cm^2  Dh=pipe.Dh cm  length_add=0 m  roughness=15e-6 m  Re_lam=2000  Re_tur=4000  shape_factor=64  Nu_lam=3.66  dynamic_compressibility=simscape.enum.onoff.off  inertia=simscape.enum.onoff.off  p0=0.101325 MPa  T0=BattTempInit degC  mdot0=0 kg/s
  Refrigerant Temperature : Subsystem  mask{T_refrig=274}
      mask prompts: T_refrig "Refrigerant nominal temperature (K)"
  Thermal Reference : fl_lib/Thermal/Thermal Elements/Thermal Reference
  B : PMIOPort  Side=Left
  A : PMIOPort  Port=2  Side=Right
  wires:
  PS-Simulink Converter/1 -> Efficiency/1  "Phref"
  Efficiency/1 -> [CmpPwr]  "RefrigPwr"
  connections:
  Pipe (TL)/RConn1 -- B/RConn1
  Controlled Temperature Source/RConn2 -- Thermal Reference/LConn1
  Mass & Energy Flow Rate Sensor (TL)/LConn1 -- A/RConn1
  Heat Flow Rate Sensor/LConn1 -- Pipe (TL)/LConn2
  Pipe (TL)/LConn1 -- Mass & Energy Flow Rate Sensor (TL)/RConn1
  Refrigerant Temperature/LConn1 -- Mass & Energy Flow Rate Sensor (TL)/RConn2
  Refrigerant Temperature/RConn1 -- Controlled Temperature Source/RConn1
  Heat Flow Rate Sensor/RConn2 -- Controlled Temperature Source/LConn1
  Heat Flow Rate Sensor/RConn1 -- PS-Simulink Converter/LConn1

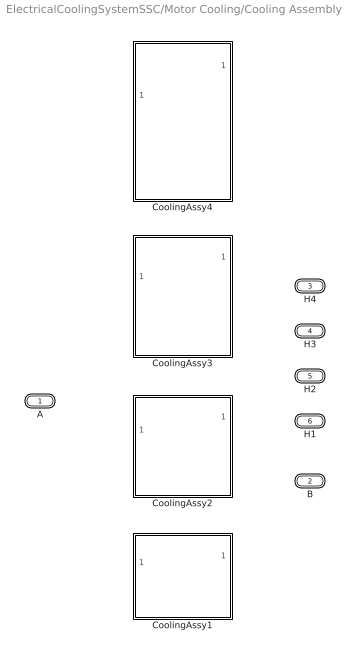
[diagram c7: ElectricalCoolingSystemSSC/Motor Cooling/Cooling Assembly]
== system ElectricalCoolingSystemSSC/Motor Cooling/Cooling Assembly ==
  CoolingAssy1 : Subsystem  VariantControl=PlntEMNum == 1
  CoolingAssy2 : Subsystem  VariantControl=PlntEMNum == 2
  CoolingAssy3 : Subsystem  VariantControl=PlntEMNum == 3
  CoolingAssy4 : Subsystem  VariantControl=PlntEMNum == 4
  A : PMIOPort  Side=Left
  B : PMIOPort  Port=2  Side=Right
  H4 : PMIOPort  Port=3  Side=Right
  H3 : PMIOPort  Port=4  Side=Right
  H2 : PMIOPort  Port=5  Side=Right
  H1 : PMIOPort  Port=6  Side=Right

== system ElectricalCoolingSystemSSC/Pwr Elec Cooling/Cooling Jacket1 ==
  Conduction : fl_lib/Thermal/Thermal Elements/Conductive Heat Transfer  thermal_type=foundation.enum.ConstantVariableTabulated.Constant  wall_geometry=foundation.enum.ConductionWallGeometry.Planar  area=0.5*2 m^2  thickness=1 mm  d_in=0.05 m  d_out=0.1 m  L=1 m  th_cond_min=10 W/(K*m)  th_cond=205 W/(m*K)  th_cond_TLU=[413, 401, 392, 383, 371, 357, 342] W/(K*m)  temp_TLU=[200, 273, 400, 600, 800, 1000, 1200] K  T_specify=off  T_priority=None  T=0 K  T_nominal_specify=off  T_nominal_value=1  T_nominal_unit=K  Q_specify=off  Q_priority=None  Q=0 W  Q_nominal_specify=off  Q_nominal_value=1  Q_nominal_unit=W
  "Mass " : fl_lib/Thermal/Thermal Elements/Thermal Mass  mass_type=foundation.enum.constant_variable.constant  mass=1 kg  sp_heat=385 J/kg/K  mass_min=1e-6 kg  num_ports=foundation.enum.numPorts2.one  m_specify=off  m_priority=High  m=1 kg  m_nominal_specify=off  m_nominal_value=1  m_nominal_unit=kg  T_specify=on  T_priority=High  T=BattTempInit degC  T_nominal_specify=off  T_nominal_value=1  T_nominal_unit=K  Q_specify=off  Q_priority=None  Q=0 W  Q_nominal_specify=off  Q_nominal_value=1  Q_nominal_unit=W
  H1 : PMIOPort  Side=Left
  T1 : PMIOPort  Port=2  Side=Right
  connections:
  Conduction/LConn1 -- T1/RConn1
  Conduction/RConn1 -- H1/RConn1 -- "Mass "/LConn1

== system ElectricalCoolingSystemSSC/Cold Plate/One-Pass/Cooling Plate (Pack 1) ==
  Battery to plate conduction : fl_lib/Thermal/Thermal Elements/Conductive Heat Transfer  thermal_type=foundation.enum.ConstantVariableTabulated.Constant  wall_geometry=foundation.enum.ConductionWallGeometry.Planar  area=0.5*2 m^2  thickness=1 mm  d_in=0.05 m  d_out=0.1 m  L=1 m  th_cond_min=10 W/(K*m)  th_cond=205 W/(m*K)  th_cond_TLU=[413, 401, 392, 383, 371, 357, 342] W/(K*m)  temp_TLU=[200, 273, 400, 600, 800, 1000, 1200] K  T_specify=off  T_priority=None  T=0 K  T_nominal_specify=off  T_nominal_value=1  T_nominal_unit=K  Q_specify=off  Q_priority=None  Q=0 W  Q_nominal_specify=off  Q_nominal_value=1  Q_nominal_unit=W
  "Plate mass " : fl_lib/Thermal/Thermal Elements/Thermal Mass  mass_type=foundation.enum.constant_variable.constant  mass=10*2 kg  sp_heat=910 J/kg/K  mass_min=1e-6 kg  num_ports=foundation.enum.numPorts2.one  m_specify=off  m_priority=High  m=1 kg  m_nominal_specify=off  m_nominal_value=1  m_nominal_unit=kg  T_specify=on  T_priority=High  T=BattTempInit degC  T_nominal_specify=off  T_nominal_value=1  T_nominal_unit=K  Q_specify=off  Q_priority=None  Q=0 W  Q_nominal_specify=off  Q_nominal_value=1  Q_nominal_unit=W
  H1 : PMIOPort  Side=Left
  T1 : PMIOPort  Port=2  Side=Right
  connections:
  T1/RConn1 -- Battery to plate conduction/LConn1
  "Plate mass "/LConn1 -- H1/RConn1 -- Battery to plate conduction/RConn1

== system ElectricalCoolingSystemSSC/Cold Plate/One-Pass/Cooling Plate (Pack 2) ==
  Battery to plate conduction : fl_lib/Thermal/Thermal Elements/Conductive Heat Transfer  thermal_type=foundation.enum.ConstantVariableTabulated.Constant  wall_geometry=foundation.enum.ConductionWallGeometry.Planar  area=0.5*2 m^2  thickness=1 mm  d_in=0.05 m  d_out=0.1 m  L=1 m  th_cond_min=10 W/(K*m)  th_cond=205 W/(m*K)  th_cond_TLU=[413, 401, 392, 383, 371, 357, 342] W/(K*m)  temp_TLU=[200, 273, 400, 600, 800, 1000, 1200] K  T_specify=off  T_priority=None  T=0 K  T_nominal_specify=off  T_nominal_value=1  T_nominal_unit=K  Q_specify=off  Q_priority=None  Q=0 W  Q_nominal_specify=off  Q_nominal_value=1  Q_nominal_unit=W
  "Plate mass " : fl_lib/Thermal/Thermal Elements/Thermal Mass  mass_type=foundation.enum.constant_variable.constant  mass=10*2 kg  sp_heat=910 J/kg/K  mass_min=1e-6 kg  num_ports=foundation.enum.numPorts2.one  m_specify=off  m_priority=High  m=1 kg  m_nominal_specify=off  m_nominal_value=1  m_nominal_unit=kg  T_specify=on  T_priority=High  T=BattTempInit degC  T_nominal_specify=off  T_nominal_value=1  T_nominal_unit=K  Q_specify=off  Q_priority=None  Q=0 W  Q_nominal_specify=off  Q_nominal_value=1  Q_nominal_unit=W
  H1 : PMIOPort  Side=Left
  T2 : PMIOPort  Port=2  Side=Right
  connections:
  T2/RConn1 -- Battery to plate conduction/LConn1
  "Plate mass "/LConn1 -- H1/RConn1 -- Battery to plate conduction/RConn1

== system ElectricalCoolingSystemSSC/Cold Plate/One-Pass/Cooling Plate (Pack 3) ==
  Battery to plate conduction : fl_lib/Thermal/Thermal Elements/Conductive Heat Transfer  thermal_type=foundation.enum.ConstantVariableTabulated.Constant  wall_geometry=foundation.enum.ConductionWallGeometry.Planar  area=0.5*2 m^2  thickness=1 mm  d_in=0.05 m  d_out=0.1 m  L=1 m  th_cond_min=10 W/(K*m)  th_cond=205 W/(m*K)  th_cond_TLU=[413, 401, 392, 383, 371, 357, 342] W/(K*m)  temp_TLU=[200, 273, 400, 600, 800, 1000, 1200] K  T_specify=off  T_priority=None  T=0 K  T_nominal_specify=off  T_nominal_value=1  T_nominal_unit=K  Q_specify=off  Q_priority=None  Q=0 W  Q_nominal_specify=off  Q_nominal_value=1  Q_nominal_unit=W
  "Plate mass " : fl_lib/Thermal/Thermal Elements/Thermal Mass  mass_type=foundation.enum.constant_variable.constant  mass=10*2 kg  sp_heat=910 J/kg/K  mass_min=1e-6 kg  num_ports=foundation.enum.numPorts2.one  m_specify=off  m_priority=High  m=1 kg  m_nominal_specify=off  m_nominal_value=1  m_nominal_unit=kg  T_specify=on  T_priority=High  T=BattTempInit degC  T_nominal_specify=off  T_nominal_value=1  T_nominal_unit=K  Q_specify=off  Q_priority=None  Q=0 W  Q_nominal_specify=off  Q_nominal_value=1  Q_nominal_unit=W
  H1 : PMIOPort  Side=Left
  T3 : PMIOPort  Port=2  Side=Right
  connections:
  T3/RConn1 -- Battery to plate conduction/LConn1
  Battery to plate conduction/RConn1 -- H1/RConn1 -- "Plate mass "/LConn1
